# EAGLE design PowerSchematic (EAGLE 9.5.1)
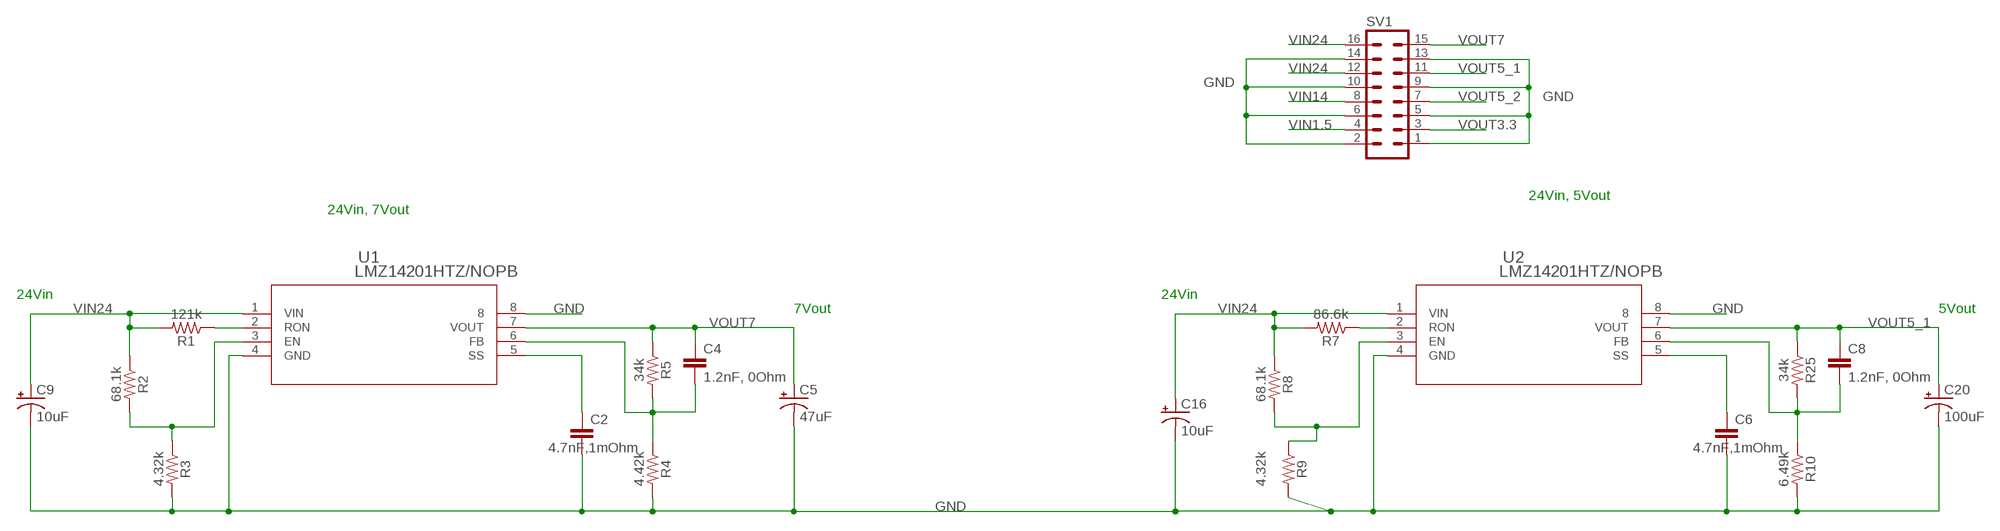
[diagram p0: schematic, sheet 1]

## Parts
C2  4.7nF,1mOhm  0.33UF/330NF-0805-50V-10%  [0805]
C4  1.2nF, 0Ohm  0.33UF/330NF-0805-50V-10%  [0805]
C5  47uF  100UF-POLAR-RADIAL-2.5MM-25V-20%  [CPOL-RADIAL-2.5MM-6.5MM]
C6  4.7nF,1mOhm  0.33UF/330NF-0805-50V-10%  [0805]
C8  1.2nF, 0Ohm  0.33UF/330NF-0805-50V-10%  [0805]
C9  10uF  10UF-POLAR-RADIAL-2.5MM-KIT-25V-20%  [CPOL-RADIAL-2.5MM-5MM-KIT]
C16  10uF  10UF-POLAR-RADIAL-2.5MM-KIT-25V-20%  [CPOL-RADIAL-2.5MM-5MM-KIT]
C20  100uF  100UF-POLAR-RADIAL-2.5MM-25V-20%  [CPOL-RADIAL-2.5MM-6.5MM]
R1  121k  0.3OHM-0805-1/8W-1%  [0805]
R2  68.1k  0.3OHM-0805-1/8W-1%  [0805]
R3  4.32k  0.3OHM-0805-1/8W-1%  [0805]
R4  4.42k  0.3OHM-0805-1/8W-1%  [0805]
R5  34k  0.3OHM-0805-1/8W-1%  [0805]
R7  86.6k  0.3OHM-0805-1/8W-1%  [0805]
R8  68.1k  0.3OHM-0805-1/8W-1%  [0805]
R9  4.32k  0.3OHM-0805-1/8W-1%  [0805]
R10  6.49k  0.3OHM-0805-1/8W-1%  [0805]
R25  34k  0.3OHM-0805-1/8W-1%  [0805]
SV1  MA08-2  [MA08-2]
U1  LMZ14201HTZ/NOPB  [TZA07A]
U2  LMZ14201HTZ/NOPB  [TZA07A]

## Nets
3_CORRECT: R8.2 R9.1 U2.3(EN)
GND: C2.2 C5.2(-) C6.2 C9.2(-) C16.2(-) C20.2(-) R3.2 R4.2 R9.2 R10.2 SV1.1 SV1.2 SV1.5 SV1.6 SV1.9 SV1.10 SV1.13 SV1.14 U1.4(GND) U1.8 U2.4(GND) U2.8
N$1: R2.2 R3.1 U1.3(EN)
N$2: R1.1 U1.2(RON)
N$5: R7.1 U2.2(RON)
N$7: C6.1 U2.5(SS)
N$8: C2.1 U1.5(SS)
N$10: C4.2 R4.1 R5.2 U1.6(FB)
N$12: C8.2 R10.1 R25.2 U2.6(FB)
VIN1.5: SV1.4
VIN14: SV1.8
VIN24: C9.1(+) C16.1(+) R1.2 R2.1 R7.2 R8.1 SV1.12 SV1.16 U1.1(VIN) U2.1(VIN)
VOUT3.3: SV1.3
VOUT5_1: C8.1 C20.1(+) R25.1 SV1.11 U2.7(VOUT)
VOUT5_2: SV1.7
VOUT7: C4.1 C5.1(+) R5.1 SV1.15 U1.7(VOUT)

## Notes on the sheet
- 24Vin, 5Vout
- 24Vin, 7Vout
- 24Vin | 24Vin
- 7Vout | 5Vout

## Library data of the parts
C2 C4 C6 C8 = SparkFun-Capacitors:0.33UF/330NF: 0.33µF/330nF ceramic capacitors; PROD_ID: CAP-08469; VALUE: 0.33µF
C5 = SparkFun-Capacitors:100UF-POLAR: 100µF polarized capacitors; PROD_ID: CAP-08439; VALUE: 100uF
C9 C16 = SparkFun-Capacitors:10UF-POLAR: 10.0µF polarized capacitors; PROD_ID: CAP-08440
C20 = SparkFun-Capacitors:100UF-POLAR: 100µF polarized capacitors; PROD_ID: CAP-08439
R1-R5 R7-R10 R25 = SparkFun-Resistors:0.3OHM: 0.3Ω resistor; PROD_ID: RES-11622; VALUE: 0.3
SV1 = con-lstb:MA08-2: PIN HEADER; OC_FARNELL: unknown; OC_NEWARK: unknown
U1 U2 = LMZ14201H:LMZ14201HTZ/NOPB; MANUFACTURER_PART_NUMBER: LMZ14201HTZNOPB; VENDOR: Texas Instruments

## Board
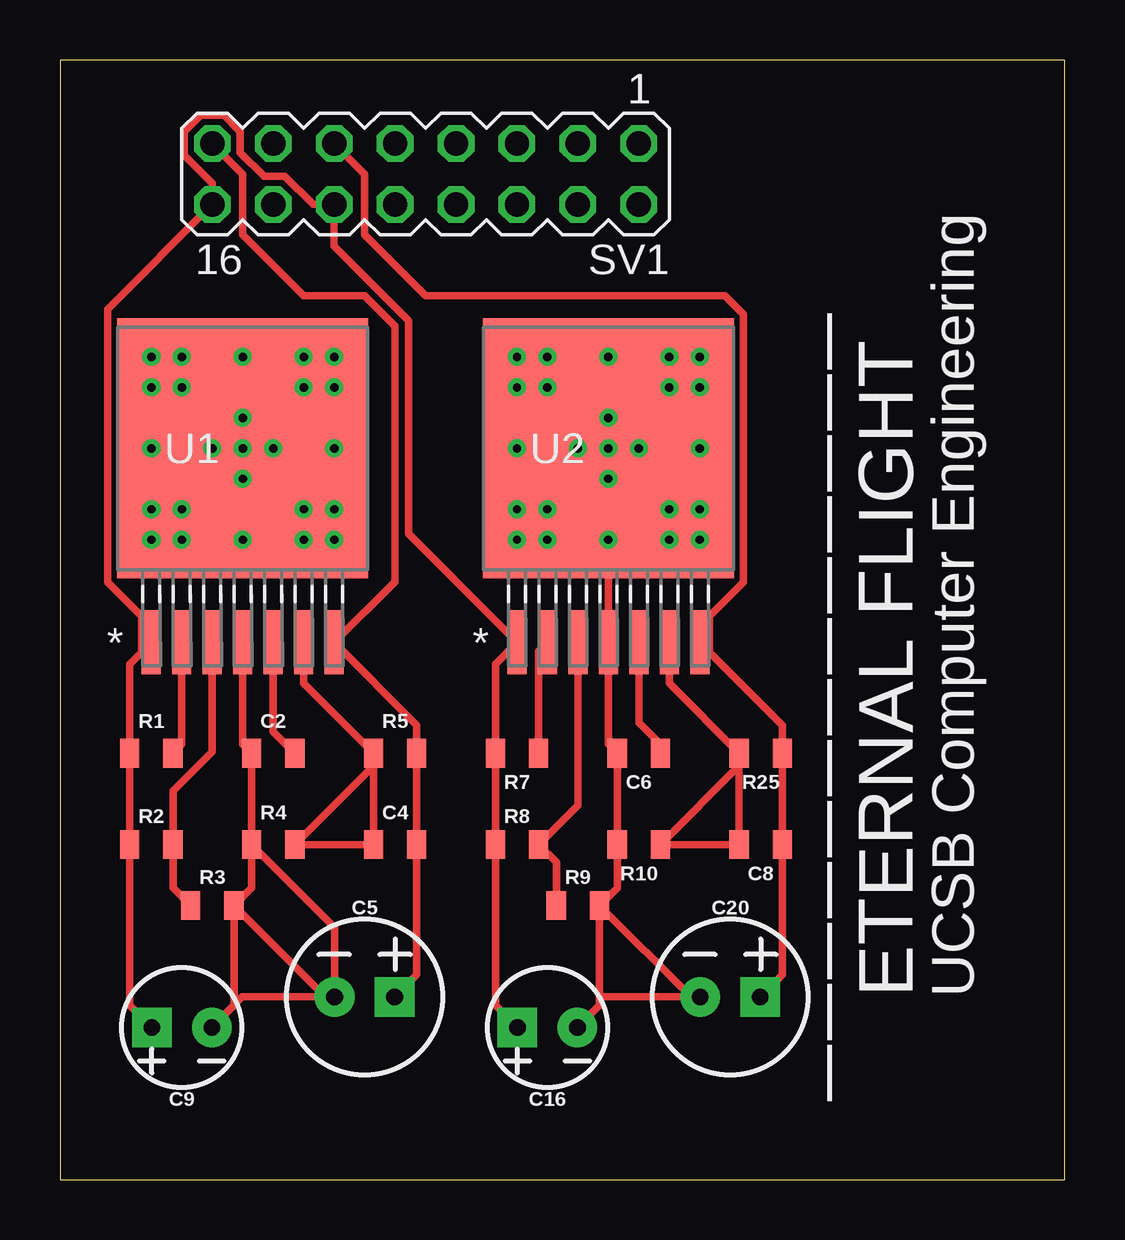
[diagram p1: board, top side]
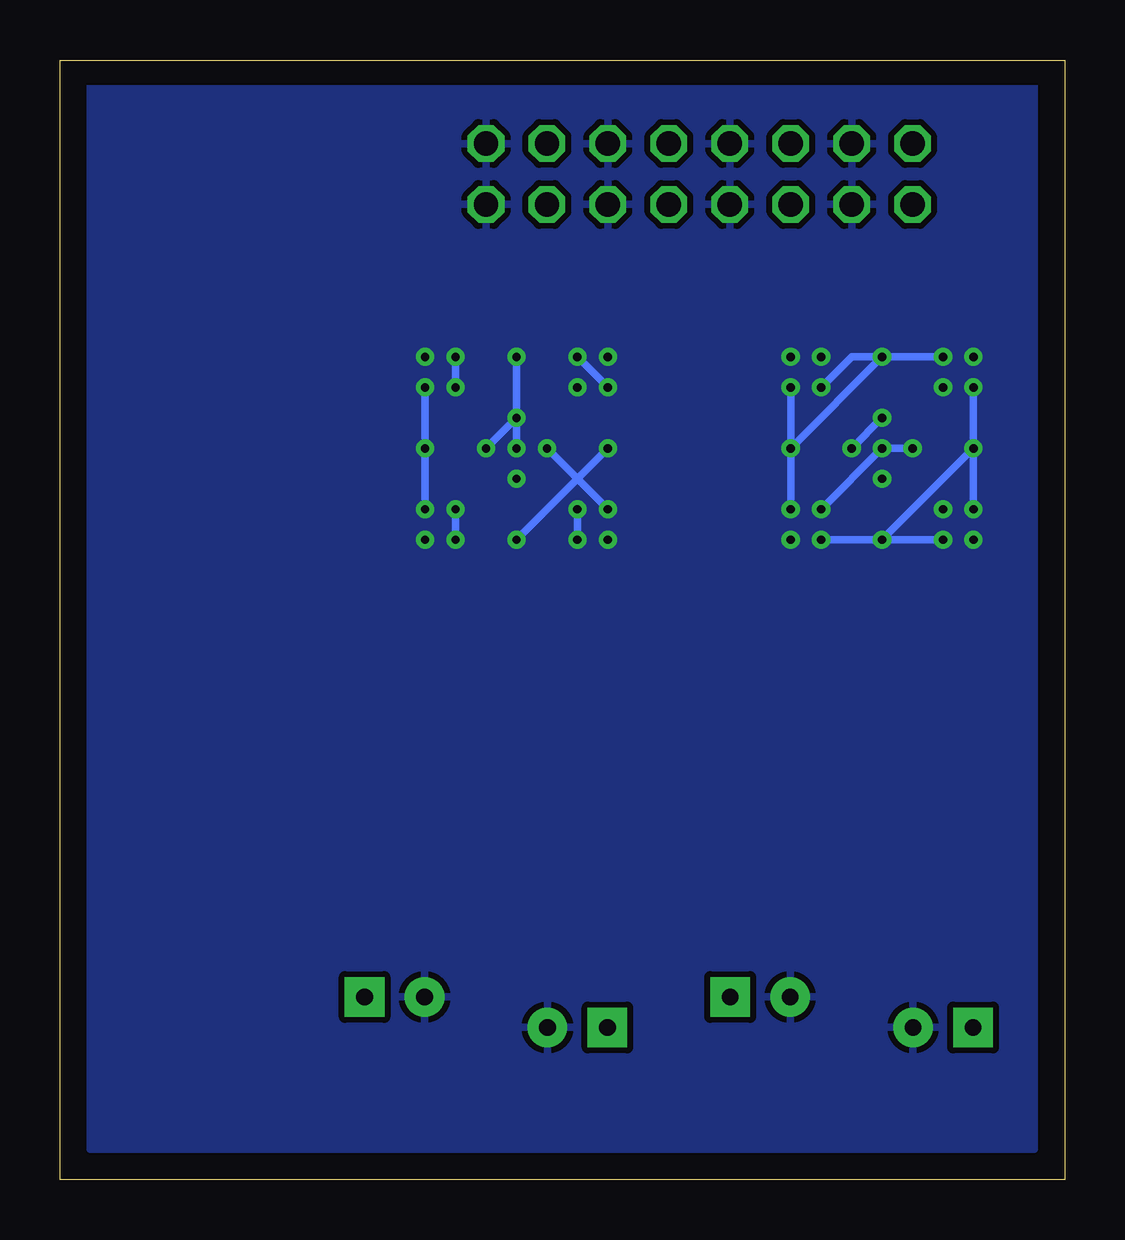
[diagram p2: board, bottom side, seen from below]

Size 41.89 x 46.66 mm. Coordinates in mm from the lower left corner, seen from the top.
Outline: 0,0 41.89,0 41.89,46.66 0,46.66 0,0
Copper layers (1*16): Top 0.035mm / dielectric 1.5mm / Bottom 0.035mm
Design rules "default *": minimum track width 12mil, minimum drill 0.35mm, track to track 10mil, track to pad 10mil, pad to pad 10mil, via to via 10mil, smd to smd 6mil, copper to edge 40mil, drill to drill 10mil, minimum pad ring 10mil, minimum via ring 8mil, stop-mask expansion 4mil, vias tented up to drill 0mil, thermal gap 10mil

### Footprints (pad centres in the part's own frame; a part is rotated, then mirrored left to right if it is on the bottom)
0805 = smd 0.8 x 1.2: 1 -0.9,0; 2 0.9,0
CPOL-RADIAL-2.5MM-6.5MM = drill 0.7 pad 1.651 square: 1 1.25,0 | drill 0.7 pad 1.651: 2 -1.25,0
CPOL-RADIAL-2.5MM-5MM-KIT = drill 0.7 pad 1.651 square: 1 1.25,0 | drill 0.7 pad 1.651: 2 -1.25,0
MA08-2 = drill 1.016 octagon: 1 -8.89,-1.27; 2 -8.89,1.27; 3 -6.35,-1.27; 4 -6.35,1.27; 5 -3.81,-1.27; 6 -3.81,1.27; 7 -1.27,-1.27; 8 -1.27,1.27; 9 1.27,-1.27; 10 1.27,1.27; 11 3.81,-1.27; 12 3.81,1.27; 13 6.35,-1.27; 14 6.35,1.27; 15 8.89,-1.27; 16 8.89,1.27
TZA07A = smd 0.787 x 2.667: 1 -3.81,-8.09; 2 -2.54,-8.09; 3 -1.27,-8.09; 4 0,-8.09; 5 1.27,-8.09; 6 2.54,-8.09; 7 3.81,-8.09 | smd 10.465 x 10.82: 8 0,0

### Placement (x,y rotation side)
C2  8.89,17.78 180 top
C4  13.97,13.97 180 top
C5  12.7,7.62 0 top
C6  24.13,17.78 180 top
C8  29.21,13.97 180 top
C9  5.08,6.35 180 top
C16  20.32,6.35 180 top
C20  27.94,7.62 0 top
R1  3.81,17.78 180 top
R2  3.81,13.97 0 top
R3  6.35,11.43 0 top
R4  8.89,13.97 180 top
R5  13.97,17.78 180 top
R7  19.05,17.78 180 top
R8  19.05,13.97 0 top
R9  21.59,11.43 0 top
R10  24.13,13.97 180 top
R25  29.21,17.78 180 top
SV1  15.24,41.91 180 top
U1  7.62,30.48 0 top
U2  22.86,30.48 0 top

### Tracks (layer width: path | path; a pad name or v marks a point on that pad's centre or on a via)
3_CORRECT
  Top 0.305: U2.3 21.59,15.61 R8.2 20.69,13.23 R9.1
GND  (via drill 0.35)
  Top 0.305: U1.4 7.62,18.15 C2.2 R4.2 | R4.2 7.99,12.17 R3.2 | R3.2 7.25,7.27 C9.2 7.6,7.62 11.06,7.62 | R4.2 11.45,10.51 C5.2 11.06,7.62 | R9.2 23.23,12.17 R10.2 C6.2 22.86,18.15 U2.4 v22.86,26.67 v26.67,30.48 | R9.2 22.49,7.62 | 22.49,7.62 22.49,7.27 C16.2 | 22.49,7.62 C20.2 26.3,7.62 R9.2 | v20.32,33.02 v19.05,34.29 | v3.81,34.29 v5.08,33.02 U1.8 | v10.16,33.02 v11.43,34.29 | v25.4,33.02 v26.67,34.29 | v3.81,26.67 v5.08,27.94 U1.8 | v20.32,27.94 v19.05,26.67 | v25.4,27.94 v26.67,26.67 | v7.62,26.67 v11.43,30.48 | v22.86,34.29 v19.05,30.48 | R3.2 11.06,7.62 | v10.16,33.02 v10.16,34.29 | U1.8 v10.16,33.02 | v10.16,33.02 v11.43,33.02 | v11.43,27.94 v10.16,26.67 | v5.08,26.67 v3.81,27.94 | v3.81,33.02 v5.08,34.29 | U1.8 v10.16,27.94 | v6.35,30.48 v7.62,31.75 | v8.89,30.48 v7.62,29.21 | U2.8 v20.32,33.02 | v20.32,33.02 v19.05,33.02 | v20.32,34.29 v20.32,33.02 | U2.8 v25.4,33.02 | v25.4,33.02 v25.4,34.29 | v26.67,33.02 v24.13,30.48 U2.8 | v26.67,27.94 v25.4,26.67 | v20.32,26.67 v22.86,29.21 v21.59,30.48 | U2.8 v21.59,30.48 | v21.59,30.48 v19.05,27.94
  Bottom 0.305: v3.81,30.48 v7.62,26.67 | v11.43,30.48 v7.62,34.29 | U2.8 v22.86,31.75 | v22.86,31.75 v22.86,34.29 | v19.05,30.48 v22.86,26.67 | v11.43,33.02 v11.43,27.94 | v10.16,26.67 v5.08,26.67 | v3.81,27.94 v3.81,33.02 | v5.08,34.29 8.89,34.29 v10.16,33.02 | v10.16,27.94 U1.8 v6.35,30.48 | v7.62,31.75 v8.89,30.48 | v19.05,33.02 v20.32,34.29 | v25.4,34.29 v25.4,33.02 | v26.67,33.02 v26.67,27.94 | v25.4,26.67 v25.4,27.94 | v20.32,26.67 v20.32,27.94 | v19.05,27.94 v21.59,30.48 | v24.13,30.48 v22.86,31.75
  other vias: 11.43,26.67 7.62,30.48 22.86,30.48
  pour Bottom: 1.27,45.72 40.64,45.72 40.64,1.27 1.27,1.27
N$1
  Top 0.305: U1.3 6.35,17.84 4.71,16.2 R2.2 4.71,12.17 R3.1
N$2
  Top 0.305: U1.2 5.08,18.15 R1.1
N$5
  Top 0.305: U2.2 19.95,22.02 R7.1
N$7
  Top 0.305: C6.1 25.03,18.15 24.13,19.05 U2.5
N$8
  Top 0.305: U1.5 8.89,18.68 C2.1
N$10
  Top 0.305: U1.6 10.16,20.69 R5.2 | R5.2 C4.2 R4.1 13.07,17.25 R5.2
N$12
  Top 0.305: R25.2 C8.2 R10.1 28.31,17.25 R25.2 | R25.2 25.4,20.69 U2.6
VIN24
  Top 0.305: U1.1 3.41,21.99 | 3.41,21.99 2.91,21.49 R1.2 R2.1 2.91,7.27 C9.1 | C16.1 18.15,7.27 R8.1 R7.2 18.15,21.49 U2.1 14.53,26.91 14.53,35.79 11.43,38.89 SV1.12 10.54,40.64 9.37,41.81 8.51,41.81 7.52,42.8 7.52,43.66 6.83,44.35 5.87,44.35 5.18,43.66 5.18,42.7 6.35,41.53 SV1.16 1.98,36.27 1.98,24.9 3.41,23.47 3.41,21.99
VOUT5_1
  Top 0.305: U2.7 27.07,21.99 | 27.07,21.99 30.11,18.95 R25.1 C8.1 30.11,8.54 C20.1 | 27.07,21.99 27.07,23.47 28.5,24.9 28.5,36.06 27.73,36.83 15.24,36.83 12.7,39.37 12.7,41.91 SV1.11
VOUT7
  Top 0.305: C5.1 14.87,8.54 C4.1 R5.1 14.87,18.95 U1.7 13.97,24.93 13.97,35.56 12.7,36.83 10.16,36.83 7.62,39.37 7.62,41.91 SV1.15

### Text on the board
tPlace: | | | | | | | | | | | | | | | | | | | | | | ETERNAL FLIGHT | UCSB Computer Engineering | | | |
